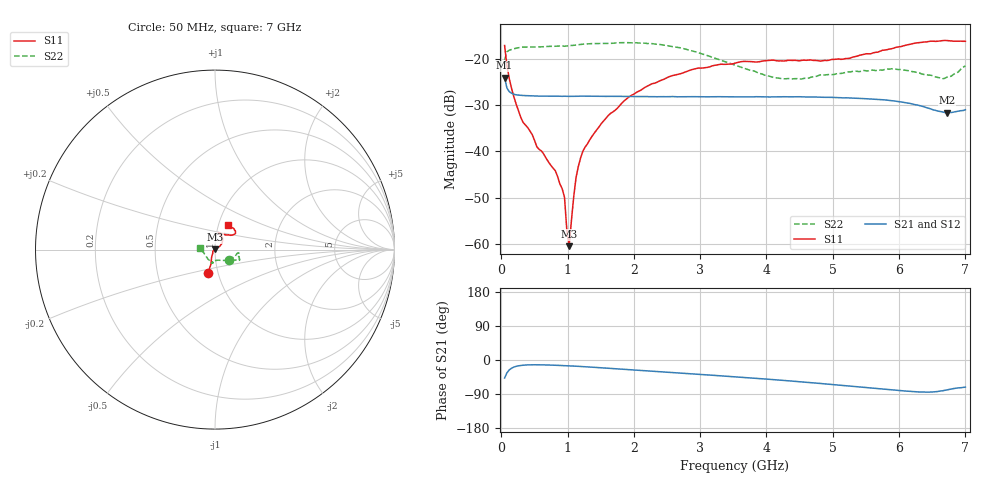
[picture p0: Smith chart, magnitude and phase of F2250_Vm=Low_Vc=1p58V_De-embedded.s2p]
! Integrated Device Technology
! Corporate Headquarters
! 6024 Silver Creek Valley Road
! San Jose, CA 95138  USA
! Phone:  1-408-284-8200
! Toll Free:  1-800-223-1366
! Webpage:  http://www.idt.com/
! Timing and RF Division
! 515 Groton Road, Suite 102
! Westford, MA 01886-6024
! Device:  F2250
! Description: Voltage Variable RF Attenuator
! Frequency:  50.0 -  6000.00 MHz
! Package:  3x3 mm Thin QFN Plastic Package: 16 pin
! Ports:  2 RF, 3 DC
!  Pin  1  = GND
!  Pin  2  = NC
!  Pin  3  = RF1  = Port 1
!  Pin  4  = NC
!  Pin  5  = GND
!  Pin  6  = GND
!  Pin  7  = GND
!  Pin  8  = GND
!  Pin  9  = NC
!  Pin 10  = RF2  = Port 2
!  Pin 11  = NC
!  Pin 12  = GND
!  Pin 13  = GND
!  Pin 14  = VCNTRL
!  Pin 15  = VDD
!  Pin 16  = VMODE
! Vcntrl:  1.580 Volts
! Vmode:  +0.000 Volts
! Vdd:  +3.30  Volts
! Current:  1.188 mA
! Data:  The device was measured on a the F2250 evaluation board which has
!  individual transmission lines to the RF pins.  Data was collected
!  using a calibrated network analyzer.  The evaluation board was
!  de-embedded using a TRL calibration technique.
!  The reference plane is the edge of the package pin.
! Misc:  SN 10
!  Action Tracker AT0258
! Date Measured:  2014-11-26
! Date:  2015-10-15  MJV
! Note:
!  Integrated Device Technology supplies this data as a sample of measured
!  data at the package pin for this product.  Your particular data for this
!  product may vary.
!  Data was taken at 25 degrees C.
!  Integrated Device Technology reserves the right to change this data at anytime.
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# GHz S dB R 50
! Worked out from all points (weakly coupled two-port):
!   201 points, 50 MHz to 7 GHz, reference 50 ohm
!   highest |S21| = -24.08 dB at 50 MHz (marker M1); lowest = -31.6 dB at 6.722 GHz (marker M2)
!   lowest |S11| = -60.4 dB at 1.023 GHz (marker M3), VSWR 1.00, Z = 50 + j0.095 ohm
!   |S11| at or under -10 dB: start of sweep to end of sweep
!   |S22| runs from -24.4 to -16.5 dB; largest |S21 - S12| = 0.00017
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0.05  -17.17 -107.1  -24.08 -47.6  -24.06 -47.6  -20.25 -38.2
0.1195  -24.27 -109.1  -27.10 -26.2  -27.11 -26.2  -18.18 -11.6
0.29325  -32.63 -121.9  -27.91 -14.4  -27.91 -14.4  -17.54 -8.5
0.5365  -39.01 -147.1  -28.05 -12.6  -28.05 -12.6  -17.48 -9.5
0.8145  -44.16 176.4  -28.10 -13.9  -28.11 -13.8  -17.32 -13.6
0.91875  -48.07 155.2  -28.12 -14.6  -28.10 -14.6  -17.25 -15.4
0.9535  -49.89 176.7  -28.10 -14.9  -28.12 -14.9  -17.33 -15.6
0.98825  -56.95 157.9  -28.12 -15.1  -28.12 -15.1  -17.25 -15.9
1.023  -60.44 92.7  -28.13 -15.4  -28.12 -15.4  -17.19 -16.0
1.0925  -49.77 39.5  -28.12 -16.0  -28.12 -16.0  -17.12 -16.8
1.12725  -45.66 35.3  -28.12 -16.3  -28.12 -16.4  -17.06 -17.4
1.2315  -39.93 30.2  -28.08 -17.4  -28.08 -17.4  -16.88 -18.9
1.6485  -31.79 36.4  -28.13 -22.0  -28.13 -22.0  -16.70 -21.6
1.9265  -28.24 37.7  -28.16 -25.2  -28.18 -25.2  -16.56 -23.0
2.37825  -24.86 44.8  -28.20 -30.5  -28.19 -30.5  -16.92 -25.0
2.93425  -22.14 58.2  -28.21 -37.1  -28.20 -37.1  -18.54 -29.2
3.525  -20.97 71.3  -28.26 -44.4  -28.24 -44.4  -21.39 -45.0
4.11575  -20.34 78.9  -28.23 -52.0  -28.21 -52.0  -24.11 -70.2
4.7065  -20.38 71.7  -28.27 -60.3  -28.30 -60.3  -23.89 -94.1
5.85325  -17.93 39.7  -29.01 -78.1  -29.01 -78.2  -22.26 -101.6
6.722  -16.09 49.6  -31.62 -78.8  -31.60 -78.9  -23.99 -156.8
7  -16.25 62.8  -31.01 -71.6  -30.98 -71.6  -21.53 175.6
